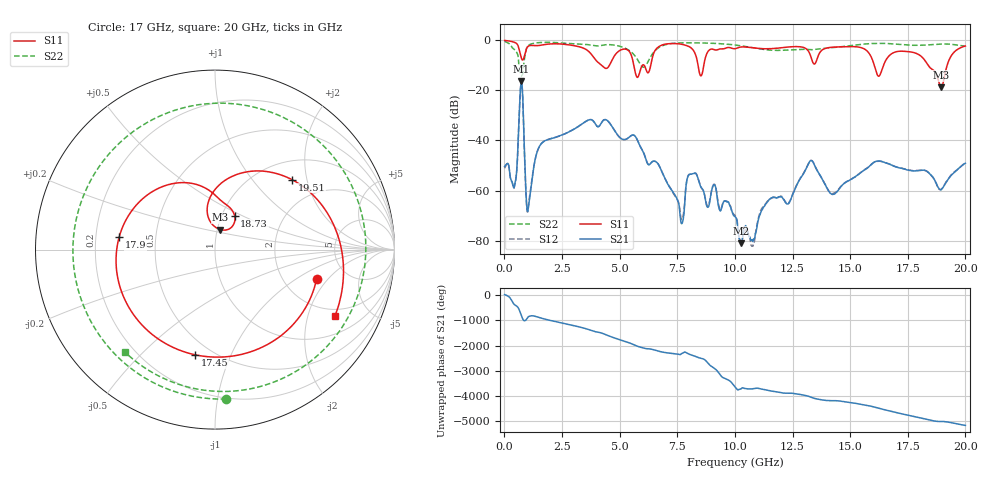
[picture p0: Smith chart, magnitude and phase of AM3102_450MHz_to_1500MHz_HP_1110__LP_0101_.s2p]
!Agilent Technologies,E8364B,MY43040894,A.07.50.67
!Agilent E8364B: A.07.50.67
!Date: Thursday, January 11, 2018 06:43:27
!Correction: S11(Full 2 Port(1,2))
!S21(Full 2 Port(1,2))
!S12(Full 2 Port(1,2))
!S22(Full 2 Port(1,2))
!S2P File: Measurements: S11, S21, S12, S22:
# Hz S  dB  R 50
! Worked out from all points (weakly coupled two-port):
!   1601 points, 10 MHz to 20 GHz, reference 50 ohm
!   highest |S21| = -16.36 dB at 734.6 MHz (marker M1); lowest = -81.0 dB at 10.25 GHz (marker M2)
!   lowest |S11| = -18.8 dB at 18.95 GHz (marker M3), VSWR 1.26, Z = 51.7 + j11.7 ohm
!   |S11| at or under -10 dB: 5.615 GHz to 5.986 GHz (371.9 MHz wide, 6.41 % of centre); 16.05 GHz to 16.45 GHz (402 MHz wide, 2.47 % of centre); 18.38 GHz to 19.21 GHz (823.4 MHz wide, 4.38 % of centre)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
!   |S22| runs from -14.1 to -0.4 dB; largest |S21 - S12| = 0.0025
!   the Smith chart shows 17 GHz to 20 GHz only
!   S11 on the Smith chart (normalised r, x): 17 GHz: 3.03, -1.52; 17.45 GHz: 0.41, -0.74; 17.9 GHz: 0.30, +0.06; 18.73 GHz: 1.15, +0.45; 19.51 GHz: 1.39, +1.63; 20 GHz: 1.68, -3.00
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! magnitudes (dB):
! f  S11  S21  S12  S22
! 10 MHz  -0.1  -50.4  -51.1  -0.4
! 447.3 MHz  -0.9  -57.5  -57.6  -3.8
! 734.6 MHz  -7.1  -16.4  -16.4  -14.1
! 1.034 GHz  -2.4  -67.2  -67.1  -2.1
! 1.572 GHz  -2.0  -41.6  -41.7  -0.9
! 3.346 GHz  -2.9  -33.6  -33.6  -1.6
! 5.77 GHz  -14.8  -39.9  -39.8  -7.6
! 6.682 GHz  -2.7  -49.6  -49.5  -3.0
! 7.694 GHz  -1.6  -73.2  -71.6  -1.0
! 8.218 GHz  -4.3  -53.2  -53.3  -1.0
! 10.01 GHz  -3.4  -70.4  -70.0  -1.9
! 10.25 GHz  -2.7  -81.0  -80.8  -2.2
! 13.34 GHz  -7.8  -48.1  -48.1  -3.8
! 14.25 GHz  -2.8  -61.6  -61.2  -3.0
! 16.68 GHz  -6.4  -49.4  -49.4  -1.3
! 17 GHz  -4.6  -50.6  -50.6  -1.6
! 17.45 GHz  -4.5  -51.7  -51.6  -1.9
! 17.9 GHz  -5.4  -52.1  -52.0  -2.0
! 18.73 GHz  -13.3  -56.9  -57.0  -1.6
! 18.95 GHz  -18.8  -59.6  -59.7  -1.5
! 19.51 GHz  -4.7  -52.9  -52.6  -1.8
! 20 GHz  -2.3  -49.1  -49.0  -2.4
